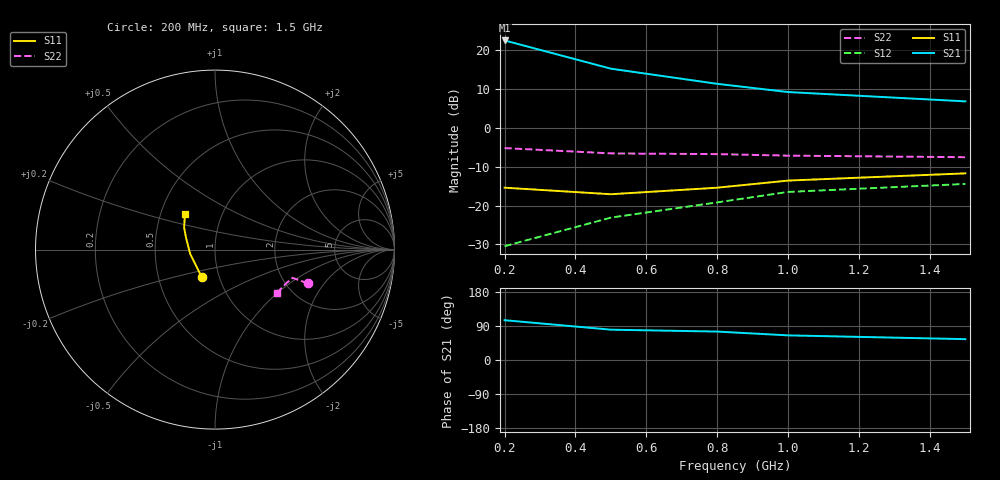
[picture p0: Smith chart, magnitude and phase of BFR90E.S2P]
!  BFR90E.S2P
!  BFR90
!  VCE=5V; IC=30mA
#  GHZ S MA R 50
!  S-PARAMETER DATA
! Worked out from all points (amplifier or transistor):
!   5 points, 200 MHz to 1.5 GHz, reference 50 ohm
!   highest |S21| = 22.5 dB at 200 MHz (marker M1)
!   |S21| within 3 dB of that: start of sweep to 323.7 MHz
!   unconditionally stable (mu >= 1): 261.3 MHz to end of sweep
!   at 200 MHz: K = 0.98, MSG = 26.5 dB, |S12| = -30.5 dB
!   at 800 MHz: K = 1.07, MAG = 13.7 dB, |S12| = -19.2 dB
!   at 1.5 GHz: K = 1.03, MAG = 9.5 dB, |S12| = -14.4 dB
0.2  0.17 -116.0  13.4 105.0  0.03 75.0  0.55 -20.0
0.5  0.14 -170.0  5.8 80.0  0.07 75.0  0.47 -20.0
0.8  0.17 160.0  3.7 75.0  0.11 75.0  0.46 -20.0
1  0.21 145.0  2.9 65.0  0.15 75.0  0.44 -25.0
1.5  0.26 130.0  2.2 55.0  0.19 70.0  0.42 -35.0
